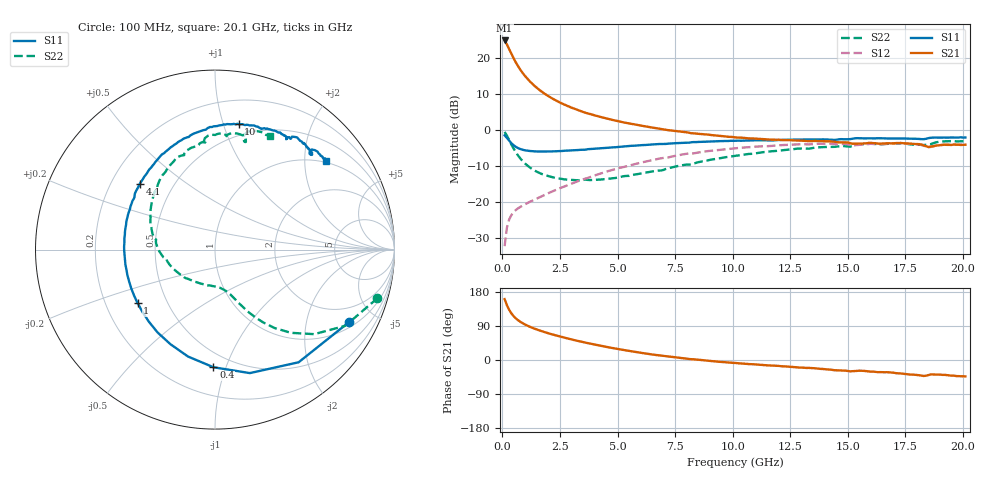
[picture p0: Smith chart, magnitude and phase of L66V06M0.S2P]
!  Infineon Technologies AG
! BFR380L3 , PF131585-7, No.6, Th 09.10.01, soldered on pcb-board, measured with PP GSG850
!  Vce=6.0 V,  Ic=6.0 mA
! Common Emitter S-Parameters:  15. November 2001
#  GHz  S  MA  R  50
! f  S11  S21  S12  S22
! GHz  Mag  Ang  Mag  Ang  Mag  Ang  Mag  Ang
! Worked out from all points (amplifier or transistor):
!   201 points, 100 MHz to 20.1 GHz, reference 50 ohm
!   highest |S21| = 24.9 dB at 100 MHz (marker M1)
!   |S21| within 3 dB of that: start of sweep to 342.4 MHz
!   unconditionally stable (mu >= 1): 2.197 GHz to 4.473 GHz; 18.49546 GHz to 18.50169 GHz
!   at 3.4 GHz: K = 1.04, MAG = 8.4 dB, |S12| = -13.9 dB
!   at 10.1 GHz: K = 0.93, MSG = 1.5 dB, |S12| = -5.0 dB
!   at 20.1 GHz: K = 0.99, MSG = 0.0 dB, |S12| = -4.0 dB
!   S11 on the Smith chart (normalised r, x): 100 MHz: 1.22, -3.53; 400 MHz: 0.39, -0.91; 1 GHz: 0.34, -0.28; 4.1 GHz: 0.32, +0.34; 10 GHz: 0.40, +1.13; 20.1 GHz: 0.96, +2.53
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0.1  0.8477 -28.6  17.52 160.8  0.02464 73.5  0.9448 -16.6
0.2  0.7817 -53.4  15.4 144.7  0.04461 63.6  0.8407 -30.3
0.3  0.715 -74.2  13.25 132.1  0.0581 55.7  0.7265 -40.4
0.4  0.6556 -90.7  11.34 122.5  0.06696 50.6  0.6275 -47.6
0.5  0.6143 -104.2  9.789 115.1  0.07342 47.6  0.5483 -52.8
0.6  0.5825 -115.3  8.547 109.2  0.07887 45.7  0.4865 -56.5
0.7  0.5617 -124.7  7.566 104.2  0.08305 44.8  0.4374 -59.3
0.8  0.5452 -132.5  6.76 100.0  0.08698 44.6  0.3984 -61.6
1  0.5243 -145.4  5.57 93.2  0.09429 44.9  0.3413 -64.9
1.2  0.514 -155.3  4.727 87.5  0.1017 45.8  0.3033 -67.6
1.4  0.5085 -163.6  4.106 82.7  0.1092 47.1  0.2757 -69.9
1.9  0.5061 -179.4  3.104 72.4  0.1296 50.0  0.2357 -75.8
2.6  0.5145 164.3  2.332 60.5  0.1614 52.3  0.2106 -85.8
3.5  0.534 147.8  1.791 47.3  0.208 52.7  0.2033 -100.7
4.1  0.5567 138.6  1.573 39.6  0.2404 51.8  0.2056 -113.4
5.1  0.5864 125.3  1.316 27.9  0.3012 47.9  0.2227 -133.2
6.8  0.6421 105.9  1.05 12.1  0.4026 38.9  0.2755 -167.8
10  0.711 79.3  0.8037 -7.5  0.5568 17.1  0.4356 144.4
10.1  0.7118 78.8  0.7949 -7.8  0.56 16.5  0.441 143.0
13.5  0.7425 60.1  0.7068 -21.8  0.6414 -6.4  0.5673 107.0
16.8  0.7665 47.9  0.6583 -32.7  0.6451 -23.7  0.6534 82.0
20.1  0.791 38.6  0.6282 -43.3  0.6337 -37.8  0.7051 64.2
